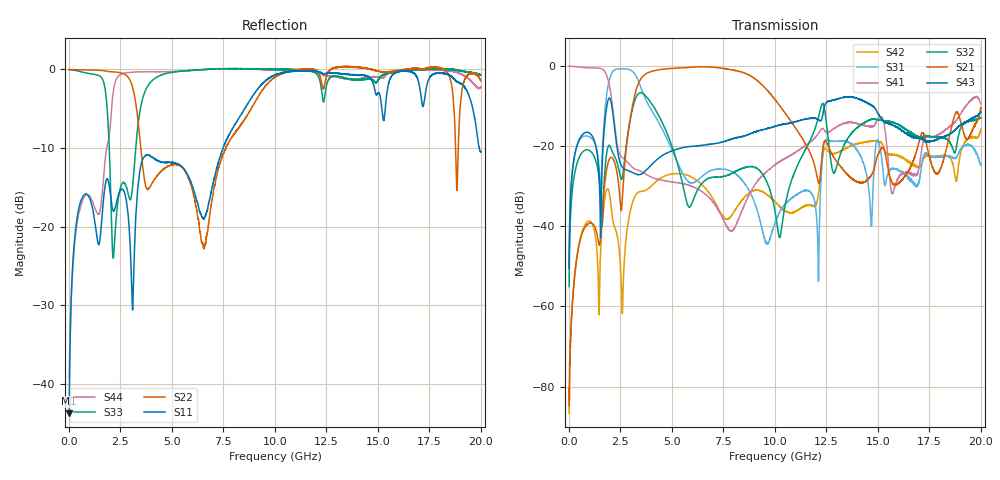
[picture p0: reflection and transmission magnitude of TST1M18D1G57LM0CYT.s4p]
# MHZ S RI R 50
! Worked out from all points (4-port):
!   3999 points, 10 MHz to 20 GHz, reference 50 ohm
!   strongest paths, dB at 10 MHz, 5.005 GHz, 10.01 GHz, 15.01 GHz, 20 GHz:
!     S43: -50.6, -21.2, -15.1, -11.9, -11.5
!     S21: -84.8, -0.7, -8.5, -22.2, -10.4
!     S32: -55.1, -20.1, -36.4, -13.5, -13.0
!     S41: -0.1, -29.0, -24.7, -13.1, -9.5
!     S31: -50.4, -21.0, -39.2, -18.6, -24.8
!     S42: -86.7, -27.0, -33.9, -18.9, -15.8
!   lowest |S11| = -43.7 dB at 10 MHz (marker M1), VSWR 1.01, Z = 50.5 - j0.409 ohm
!   |S11| at or under -10 dB: start of sweep to 7.491 GHz; 19.91813 GHz to end of sweep
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10  0.00509 -0.00405  -3.2e-05 5.72e-05  6.39e-05 0.00297  0.9847 -0.0138
    -1.26e-05 5.63e-05  0.9955 -0.00749  2.97e-05 0.00175  2.47e-05 5.46e-05
    6.4e-05 0.003  1.57e-05 0.00177  0.9945 -0.0255  5.91e-05 0.00291
    0.9871 -0.0125  -8e-06 4.57e-05  6.77e-05 0.00296  0.0108 -0.000729
1430  0.0177 0.075  -0.0039 0.00506  0.062 0.0238  -0.3451 -0.867
      -0.00391 0.005  0.5071 -0.8457  0.0442 -0.0157  0.00116 -0.00144
      0.0619 0.024  0.0442 -0.0154  -0.9061 -0.1341  -0.0115 -0.0563
      -0.3462 -0.8687  0.00115 -0.00143  -0.0118 -0.0563  -0.0447 -0.1116
3735  -0.0827 -0.2721  -0.541 0.5791  -0.0784 -0.3714  -0.0266 0.0358
      -0.5392 0.5781  -0.1733 0.0467  0.4098 -0.09  -0.0054 0.0276
      -0.0787 -0.3708  0.4096 -0.0899  0.305 -0.6791  -0.0493 -0.00468
      -0.0266 0.0356  -0.00547 0.0275  -0.0492 -0.00475  -0.4777 -0.8382
6325  -0.1267 0.0181  0.9674 0.027  0.0223 -0.0322  0.0284 -0.00123
      0.9685 0.0281  0.0956 0.0344  0.0107 0.0289  0.0329 0.0129
      0.0222 -0.032  0.0107 0.0286  -0.8952 -0.4312  -0.0361 0.0936
      0.0283 -0.00121  0.0329 0.0127  -0.0361 0.094  -0.9489 -0.2972
10225  -0.5271 -0.7816  -0.294 -0.1198  0.000463 0.0146  -0.0367 0.0509
       -0.2971 -0.1197  0.8581 -0.343  0.00116 0.00709  0.0116 0.0133
       0.000416 0.0149  0.00122 0.00719  -0.9848 -0.1721  -0.0472 0.178
       -0.0375 0.0513  0.0115 0.0134  -0.0472 0.1762  -0.9195 -0.3633
12300  -0.8814 -0.3356  -0.0585 -0.0556  -0.0672 -3.75e-05  -0.0109 0.1647
       -0.0585 -0.0564  0.1722 -0.7641  0.000822 0.3378  0.00066 -0.0686
       -0.0675 3.57e-05  0.00397 0.3367  -0.6734 0.0327  -0.1106 0.1975
       -0.00982 0.1652  -0.000368 -0.0686  -0.1098 0.1984  -0.9063 -0.2179
20000  0.2399 0.177  0.286 0.0955  0.00709 -0.0556  0.3119 -0.0744
       0.2855 0.0956  -0.7626 -0.3604  0.00455 0.2199  -0.0338 0.1528
       0.00592 -0.0569  0.0107 0.2224  -0.8369 0.3769  0.0824 0.2472
       0.3238 -0.0821  -0.032 0.1595  0.0816 0.2541  -0.7359 -0.2225
